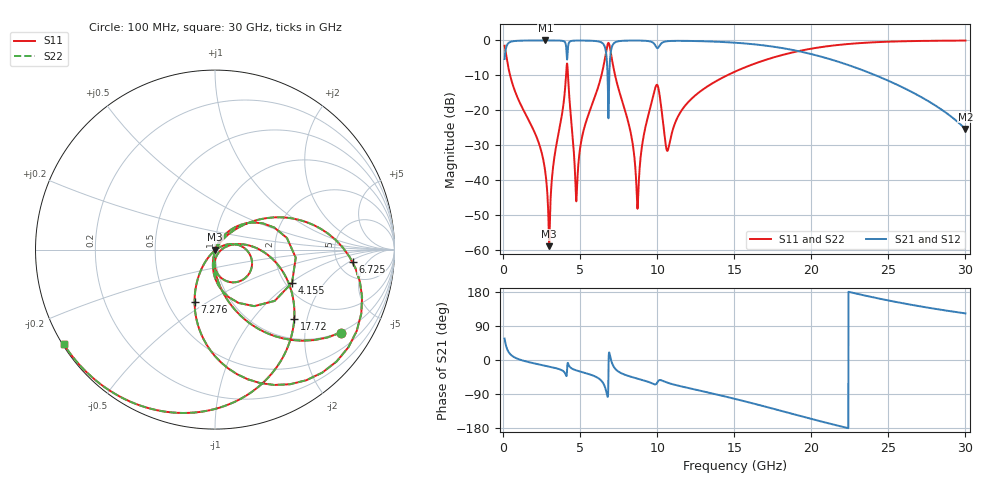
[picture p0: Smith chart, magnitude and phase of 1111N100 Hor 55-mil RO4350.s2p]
# GHz S MA R 50
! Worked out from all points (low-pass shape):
!   3201 points, 100 MHz to 30 GHz, reference 50 ohm
!   highest |S21| = -0.01 dB at 2.744 GHz (marker M1); lowest = -25.3 dB at 30 GHz (marker M2)
!   |S21| within 3 dB of the highest: 154.8 MHz to 4.115 GHz (3.961 GHz wide, 185 % of centre); 7.001 GHz to 19.11 GHz (12.11 GHz wide, 92.8 % of centre)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
!   lowest |S11| = -58.8 dB at 2.987 GHz (marker M3), VSWR 1.00, Z = 50.1 - j0.0554 ohm
!   |S11| at or under -10 dB: 457.9 MHz to 4.085 GHz (3.627 GHz wide, 160 % of centre); 4.214 GHz to 6.383 GHz (2.169 GHz wide, 40.9 % of centre); 7.271 GHz to 14.53 GHz (7.255 GHz wide, 66.6 % of centre)
!   |S22| runs from -58.8 to 0.0 dB; largest |S21 - S12| = 0
!   S11 on the Smith chart (normalised r, x): 100 MHz: 0.97, -3.05; 4.155 GHz: 2.17, -1.02; 6.725 GHz: 6.86, -2.36; 7.276 GHz: 0.68, -0.44; 17.72 GHz: 1.42, -1.67; 30 GHz: 0.00, -0.29
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0.1  0.84 -33.4  0.5423 56.6  0.5423 56.6  0.84 -33.4
0.6139062  0.2385 -79.7  0.9706 10.2  0.9706 10.2  0.2385 -79.7
2.744281  0.01304 -101.0  0.9986 -15.2  0.9986 -15.2  0.01304 -101.0
2.987219  0.001152 -28.7  0.9985 -17.4  0.9985 -17.4  0.001152 -28.7
4.155188  0.4672 -23.2  0.5324 -24.7  0.5324 -24.7  0.4672 -23.2
4.715813  0.00698 -66.7  0.9941 -26.9  0.9941 -26.9  0.00698 -66.7
5.089563  0.03809 53.2  0.9952 -31.5  0.9952 -31.5  0.03809 53.2
6.472437  0.3852 27.8  0.905 -59.6  0.905 -59.6  0.3852 27.8
6.724719  0.7698 -5.2  0.5499 -88.2  0.5499 -88.2  0.7698 -5.2
6.948969  0.7649 -73.7  0.5638 10.0  0.5638 10.0  0.7649 -73.7
7.276  0.3126 -111.4  0.9396 -23.1  0.9396 -23.1  0.3126 -111.4
8.275781  0.04881 -130.7  0.9951 -43.9  0.9951 -43.9  0.04881 -130.7
8.714937  0.004033 -64.3  0.9951 -49.0  0.9951 -49.0  0.004033 -64.3
9.247531  0.05891 24.9  0.9871 -55.2  0.9871 -55.2  0.05891 24.9
10.06978  0.2121 -59.4  0.7872 -55.4  0.7872 -55.4  0.2121 -59.4
10.68647  0.02686 -29.2  0.9757 -60.2  0.9757 -60.2  0.02686 -29.2
11.94787  0.1268 13.9  0.9843 -73.2  0.9843 -73.2  0.1268 13.9
15.05  0.3584 -13.3  0.9274 -102.6  0.9274 -102.6  0.3584 -13.3
17.72231  0.5862 -41.1  0.8027 -130.6  0.8027 -130.6  0.5862 -41.1
20.03956  0.7649 -66.3  0.6349 -155.8  0.6349 -155.8  0.7649 -66.3
25.01978  0.9594 -113.5  0.2644 157.0  0.2644 157.0  0.9594 -113.5
30  0.9943 -147.9  0.0542 123.0  0.0542 123.0  0.9943 -147.9
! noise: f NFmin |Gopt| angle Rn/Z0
0.1  0.0008855  0.7993  2.895  0.0009135
3.417  0.01126  0.5301  19.49  0.004112
6.743  0.1691  0.9239  38.13  0.4399
10.06  0.2178  0.9132  56.18  0.4307
13.39  0.03519  0.4637  69.02  0.007984
16.7  0.04356  0.4791  79.77  0.00911
20.03  0.06323  0.5786  93.5  0.01383
23.35  0.1045  0.7133  110.7  0.02464
26.67  0.2103  0.8456  129.7  0.05393
30  0.6614  0.9479  148.5  0.2121
